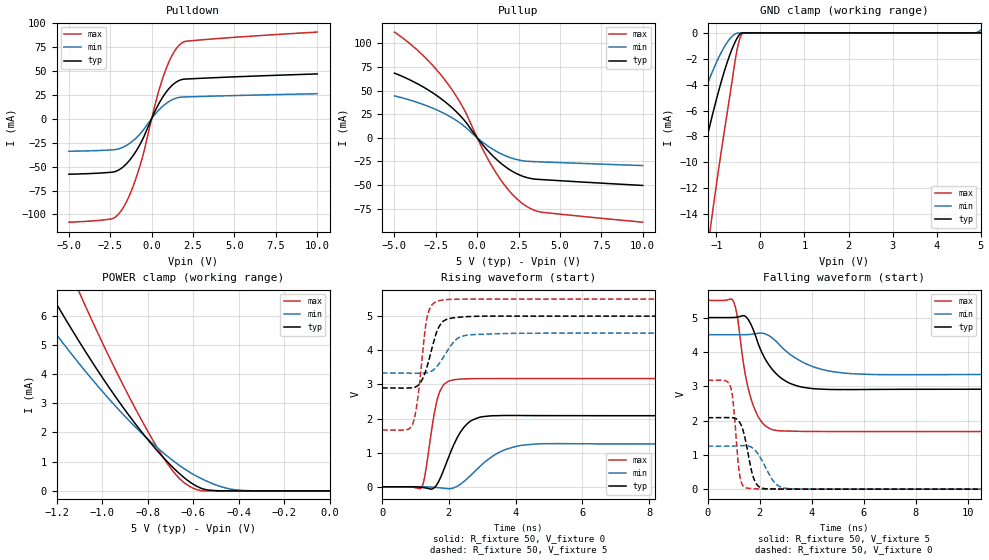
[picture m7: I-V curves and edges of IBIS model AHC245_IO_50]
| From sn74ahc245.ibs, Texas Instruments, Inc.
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[Model]   AHC245_IO_50
Model_type  I/O
Vinl = 1.65
Vinh = 3.85
Enable   Active-Low
|Vref =   0.0
|Rref =   1000
Cref =   50p
Vmeas =   2.5
| variable   typ   min   max
C_comp   2.47pF   2.32pF   2.54pF
| C_pullup   3.19pF   2.22pF   3.57pF
| C_pulldown   3.45pF   2.47pF   4.44pF
| C_tri-state   2.47pF   2.32pF   2.54pF
[Temperature Range]   40   100   -40
| Ambient temperature   25   85   -40
[Voltage range]   5   4.5   5.5
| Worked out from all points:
|   slope of the pulldown table from 0 to 0.75 V, typ, clamps not added: 30.5 ohm
|   slope of the pullup table from 0 to 0.75 V, typ, clamps not added: 47.9 ohm
|   GND clamp passes 1 mA (typ) near -0.62 V on its own axis
|   POWER clamp passes 1 mA (typ) near -0.71 V on its own axis
|   rising waveform, R_fixture 50, V_fixture 0: 20-80 % time 580ps typ, 932ps min, 314ps max; typ from 0.001 V to 2.08 V
|   falling waveform, R_fixture 50, V_fixture 5: 20-80 % time 901ps typ, 1.36ns min, 557ps max; typ from 5 V to 2.91 V
|   rising waveform, R_fixture 50, V_fixture 5: 20-80 % time 373ps typ, 493ps min, 261ps max; typ from 2.9 V to 5 V
|   falling waveform, R_fixture 50, V_fixture 0: 20-80 % time 350ps typ, 553ps min, 213ps max; typ from 2.08 V to 0.001 V
[GND Clamp]
| AHC245_IO_50
|   Voltage   I(typ)   I(min)   I(max)
-5V       -78.81mA   -50.12mA   -136.4mA
-2.23V    -24.94mA   -14.78mA   -46.01mA
-1.68V    -15.38mA   -8.616mA   -29.73mA
-1.625V   -14.47mA   -8.037mA   -28.17mA
-1.165V   -7.379mA   -3.614mA   -15.78mA
-1.115V   -6.679mA   -3.193mA   -14.53mA
-815mV    -2.915mA   -1.055mA   -7.477mA
-555mV    -563.9uA   -54.26uA   -1.741mA
-470mV    -115.1uA   -10.44uA   -463.8uA
-380mV    -131.6nA   -4.409uA   -157.9nA
4.8V      69.01pA    1.353uA    61.5pA
5V        83.23pA    205.6uA    67.5pA
[POWER Clamp]
| AHC245_IO_50
|   Voltage   I(typ)   I(min)   I(max)
-5V       82.21mA    63.82mA    114.6mA
-1.33V    8.18mA     6.73mA     11.09mA
-1.225V   6.73mA     5.607mA    9.068mA
-1.195V   6.33mA     5.298mA    8.509mA
-1.095V   5.044mA    4.304mA    6.709mA
-940mV    3.214mA    2.893mA    4.131mA
-815mV    1.912mA    1.892mA    2.265mA
-715mV    1.013mA    1.202mA    962.5uA
-640mV    460.2uA    766.3uA    287.9uA
-550mV    55.02uA    371.4uA    480.3nA
-425mV    660.6nA    49.59uA    160.7pA
-84.45fV  83.23pA    213.2pA    91.79pA
[Pulldown]
| AHC245_IO_50
|   Voltage   I(typ)   I(min)   I(max)
-5V       -57.99mA   -34.05mA   -108mA
-2.425V   -55.91mA   -32.62mA   -104.6mA
-1.74V    -50.55mA   -29.88mA   -93.42mA
-1.25V    -41.58mA   -24.76mA   -76.28mA
-755mV    -28.45mA   -16.97mA   -51.94mA
-455mV    -18.23mA   -10.68mA   -33.5mA
270mV     10.08mA    5.856mA    18.83mA
755mV     24.71mA    14.21mA    46.51mA
1.27V     35.25mA    19.95mA    67.09mA
1.78V     40.53mA    22.41mA    78.37mA
3.02V     42.08mA    23.13mA    82.17mA
10V       46.62mA    25.94mA    90.25mA
[Pullup]
| AHC245_IO_50
|   Voltage   I(typ)   I(min)   I(max)
-5V       68.44mA    44.34mA    111.9mA
-3.3V     54.16mA    35.52mA    87.59mA
-2.535V   45.75mA    30.19mA    73.59mA
-1.83V    36.49mA    24.21mA    58.38mA
-780mV    18.48mA    12.21mA    29.59mA
295mV     -6.561mA   -4.214mA   -10.71mA
1.07V     -21.3mA    -13.46mA   -35.18mA
1.89V     -32.92mA   -20.33mA   -55.22mA
2.705V    -40.38mA   -24.16mA   -69.16mA
3.295V    -43.25mA   -25.1mA    -75.51mA
3.89V     -44.2mA    -25.52mA   -78.76mA
10V       -50.44mA   -29.38mA   -89.32mA
[Ramp]
| AHC245_IO_50
| variable   typ   min   max
dV/dt_r   1.29/6.12E-10   0.79/1.01E-09   1.94/3.21E-10
dV/dt_f   1.29/9.33E-10   0.73/1.40E-09   2.32/5.66E-10
R_load = 50
[Rising Waveform]
| AHC245_IO_50
R_fixture =   50
C_fixture =   0
L_fixture =   0
V_fixture =   0
V_fixture_min = 0
V_fixture_max = 0
|   Time   V(typ)   V(min)   V(max)
0s        530.9uV    719.4uV    332.3uV
1.19ns    -15.77mV   777.2uV    -12.46mV
1.29ns    -31.06mV   -270.6uV   368.7mV
1.57ns    -21.07mV   -16.05mV   2.175V
1.71ns    187.4mV    -28.52mV   2.74V
2.365ns   1.625V     87.52mV    3.157V
2.74ns    1.971V     413.9mV    3.168V
3.53ns    2.086V     1.02V      3.17V
4.78ns    2.086V     1.262V     3.172V
49.99ns   2.082V     1.253V     3.172V
[Falling Waveform]
| AHC245_IO_50
R_fixture =   50
C_fixture =   0
L_fixture =   0
V_fixture =   5
V_fixture_min = 4.5
V_fixture_max = 5.5
|   Time   V(typ)   V(min)   V(max)
0s        5V         4.5V       5.5V
990ps     5.002V     4.499V     5.478V
1.15ns    5.015V     4.498V     4.986V
1.46ns    5.03V      4.501V     3.302V
1.73ns    4.694V     4.519V     2.494V
2.155ns   3.877V     4.537V     1.89V
2.745ns   3.287V     4.223V     1.702V
4.16ns    2.922V     3.541V     1.681V
6.295ns   2.906V     3.342V     1.68V
49.99ns   2.908V     3.34V      1.676V
[Rising Waveform]
| AHC245_IO_50
R_fixture =   50
C_fixture =   0
L_fixture =   0
V_fixture =   5
V_fixture_min = 4.5
V_fixture_max = 5.5
|   Time   V(typ)   V(min)   V(max)
0s        2.897V     3.333V     1.664V
910ps     2.901V     3.327V     1.812V
1.06ns    2.959V     3.327V     2.523V
1.28ns    3.317V     3.334V     4.522V
1.365ns   3.579V     3.345V     5.032V
1.645ns   4.558V     3.529V     5.432V
1.905ns   4.892V     3.901V     5.482V
2.38ns    4.974V     4.405V     5.497V
4.05ns    5V         4.497V     5.5V
49.99ns   5V         4.5V       5.5V
[Falling Waveform]
| AHC245_IO_50
R_fixture =   50
C_fixture =   0
L_fixture =   0
V_fixture =   0
V_fixture_min = 0
V_fixture_max = 0
|   Time   V(typ)   V(min)   V(max)
0s        2.082V     1.253V     3.172V
860ps     2.084V     1.254V     3.026V
975ps     2.079V     1.256V     2.586V
1.245ns   1.932V     1.264V     365.2mV
1.595ns   884.9mV    1.252V     23.48mV
1.775ns   313.7mV    1.17V      14.32mV
2ns       57.7mV     955.7mV    6.159mV
2.615ns   6.133mV    163mV      679.6uV
3.3ns     1.129mV    7.146mV    -58.34uV
49.99ns   529.6uV    729.9uV    332.1uV
